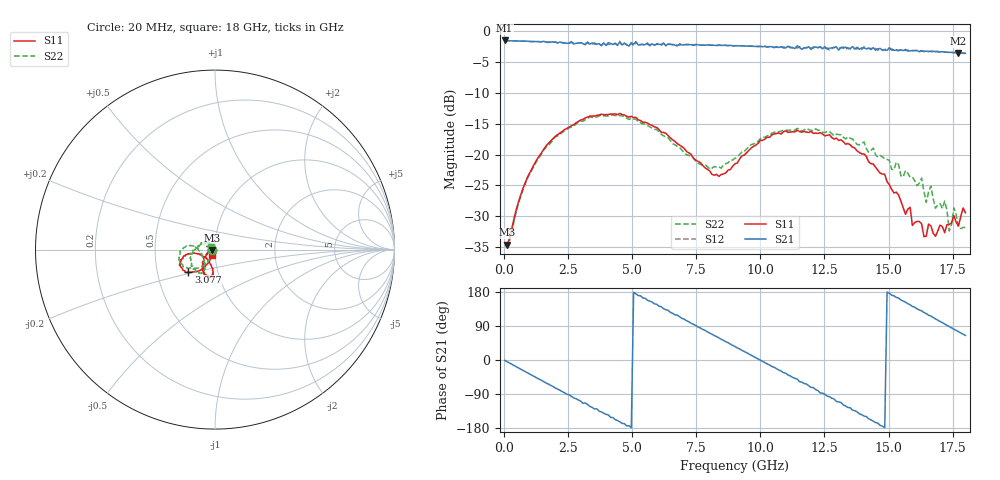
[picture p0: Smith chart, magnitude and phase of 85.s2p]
!Agilent Technologies,N5230A,US43500223,A.07.50.48
!Agilent N5230A: A.07.50.48
!Date: Sunday, January 17, 2016 19:08:55
!Correction: S11(Full 2 Port(1,2))
!S21(Full 2 Port(1,2))
!S12(Full 2 Port(1,2))
!S22(Full 2 Port(1,2))
!S2P File: Measurements: S11, S21, S12, S22:
# Hz S  RI  R 50
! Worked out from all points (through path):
!   201 points, 20 MHz to 18 GHz, reference 50 ohm
!   highest |S21| = -1.47 dB at 20 MHz (marker M1); lowest = -3.6 dB at 17.73 GHz (marker M2)
!   group delay of S21, straight-line fit = 101 ps
!   lowest |S11| = -34.6 dB at 109.9 MHz (marker M3), VSWR 1.04, Z = 48.2 - j0.447 ohm
!   |S11| at or under -10 dB: start of sweep to end of sweep
!   |S22| runs from -34.8 to -13.6 dB; largest |S21 - S12| = 0.042
!   S11 on the Smith chart (normalised r, x): 20 MHz: 0.96, -0.00; 3.077 GHz: 0.72, -0.19; 18 GHz: 0.97, -0.06
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2e7  -0.0193 -0.000248  0.8439 -0.0122  0.8428 -0.0132  -0.0184 0.000179
1.099e8  -0.0181 -0.00463  0.8382 -0.0621  0.8386 -0.0623  -0.0175 -0.00467
7.392e8  -0.0228 -0.0484  0.7374 -0.3861  0.7367 -0.3869  -0.0262 -0.0453
1.5483e9  -0.0572 -0.0951  0.4508 -0.6971  0.4495 -0.6958  -0.0628 -0.0893
3.0766e9  -0.148 -0.1241  -0.327 -0.7249  -0.3142 -0.7398  -0.1576 -0.1001
4.515e9  -0.1984 -0.0859  -0.7784 -0.2376  -0.7931 -0.2485  -0.2051 -0.0378
5.1443e9  -0.1921 -0.0583  -0.8154 0.0745  -0.8247 0.0602  -0.1945 -0.00717
6.0433e9  -0.1576 -0.0272  -0.6189 0.4842  -0.6099 0.4953  -0.1524 0.0199
7.4817e9  -0.0862 -0.0263  -0.0143 0.7843  -0.00467 0.7801  -0.0883 -0.00543
8.3807e9  -0.0467 -0.0475  0.4077 0.6592  0.4085 0.653  -0.0673 -0.0429
9.01e9  -0.0277 -0.0797  0.623 0.4448  0.6229 0.4416  -0.0567 -0.0743
1.03585e10  -0.0131 -0.1376  0.7331 -0.1708  0.7289 -0.1796  -0.0698 -0.1249
1.20666e10  -0.054 -0.1387  0.2197 -0.7131  0.1927 -0.7053  -0.1259 -0.092
1.31454e10  -0.0714 -0.111  -0.281 -0.6852  -0.2946 -0.6748  -0.1378 -0.044
1.40444e10  -0.0707 -0.0727  -0.6217 -0.3901  -0.6334 -0.4011  -0.1266 -0.0067
1.50333e10  -0.0499 -0.0278  -0.7356 0.0496  -0.7079 0.0558  -0.0864 0.024
1.63818e10  -0.0193 -0.00974  -0.3953 0.5588  -0.3937 0.5708  -0.0365 0.0345
1.71909e10  -0.0142 -0.0185  -0.0582 0.6794  -0.0504 0.6758  -0.0367 0.0204
1.73707e10  -0.0112 -0.0247  0.0213 0.6757  0.0288 0.674  -0.0184 0.0156
1.75505e10  -0.0141 -0.0288  0.1003 0.6673  0.1109 0.6605  -0.0309 0.0204
1.77303e10  -0.0118 -0.0236  0.1761 0.6399  0.1861 0.6426  -0.0254 0.00318
1.8e10  -0.0154 -0.0301  0.2823 0.6021  0.2923 0.5926  -0.0219 0.0135
